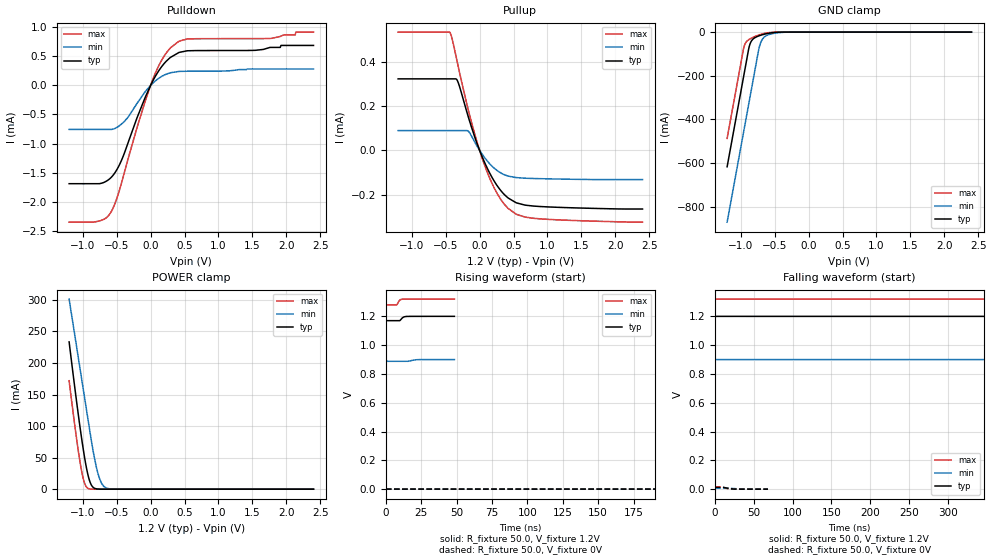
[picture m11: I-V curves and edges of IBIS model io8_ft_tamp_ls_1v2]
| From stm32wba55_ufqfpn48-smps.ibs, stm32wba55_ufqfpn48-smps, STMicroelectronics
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[Model]   io8_ft_tamp_ls_1v2
Model_type I/O
Polarity   Non-Inverting
Enable   Active-Low
| CAP_THRESHOLD on pad IOFT is "UDTCAPC" :
| Rising=30.0% of vddiom   Falling=70.0% of vddiom
| C_comp min and max val. don't necessarily correlate with the min and max pvt
| but are the smallest and greatest pad capacitance found.
| var   typ   min   max
C_comp   4.69416pF  4.27704pF  4.82289pF
|C_comp_pullup   2.95769pF  2.69399pF  2.96399pF
|C_comp_pulldown   1.73647pF  1.58305pF  1.85890pF
Vinl = 450.0mV
Vinh = 660.0mV
Vmeas = 600.0mV   | Reference voltage for timing measurements
Cref  = 50.0pF   | Timing specification test load capacitance value
Rref  = 1.0MOhm   | Timing specification test load resistance value
Vref  = 660.0mV   | Timing specification test load voltage
[Model Spec]
| TIME_THRESHOLD on pin ZIV33SW is "CMOS" :
| Rising=50.0% of VDDV33SW   Falling=50.0% of VDDV33SW
Vinl 436.50000mV 342.50000mV 466.50000mV
Vinh 753.50000mV 549.50000mV 839.50000mV
| variable   typ   min   max
[Temperature Range] 25.0 140.0 -40.0
| variable   typ   min   max
[Voltage Range] 1.2V 900.0mV 1.32V
| variable   typ   min   max
[POWER Clamp Reference] 1.2V 900.0mV 1.32V
| variable   typ   min   max
[GND Clamp Reference] 0V 0V 0V
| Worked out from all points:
|   slope of the pulldown table from 0 to 0.18 V, typ, clamps not added: 517 ohm
|   slope of the pullup table from 0 to 0.18 V, typ, clamps not added: 1.49 kohm
|   GND clamp passes 1 mA (typ) near -0.47 V on its own axis
|   POWER clamp passes 1 mA (typ) near -0.81 V on its own axis
[POWER Clamp]
-1.2V     233.4mA    301.3mA    171.8mA
-1.06V    114.5mA    205.3mA    57.35mA
-1.02V    83.5mA     177.8mA    30.99mA
-980mV    55.21mA    150.4mA    11.87mA
-920mV    21.5mA     109.2mA    1.195mA
-870mV    6.13mA     75.36mA    121.6uA
-820mV    1.189mA    45.7mA     11.82uA
-770mV    199.4uA    22.94mA    1.144uA
-730mV    46.68uA    11.1mA     176.6nA
-680mV    7.557uA    3.666mA    17.16nA
-510mV    15.46nA    46.13uA    134.2pA
2.4V      0A         0A         0A
[GND Clamp]
-1.2V     -616.6mA   -870.4mA   -486.7mA
-960mV    -208.6mA   -462.4mA   -78.75mA
-940mV    -174.6mA   -428.4mA   -56.97mA
-880mV    -73.49mA   -326.4mA   -34.53mA
-850mV    -45.28mA   -275.4mA   -29.09mA
-810mV    -29.66mA   -207.4mA   -23mA
-730mV    -17.09mA   -73.72mA   -13.06mA
-690mV    -13mA      -37.99mA   -9.157mA
-640mV    -8.81mA    -19.57mA   -5.341mA
-520mV    -2.385mA   -6.292mA   -748.7uA
-300mV    -8.501uA   -273.8uA   -150.7nA
2.4V      1.845nA    2.377uA    739.2pA
| variable   typ   min   max
[Pullup Reference] 1.2V 900.0mV 1.32V
| variable   typ   min   max
[Pulldown Reference] 0V 0V 0V
[Pullup]
-1.2V     323uA      89.11uA    534.5uA
-440mV    323uA      89.11uA    534uA
-400mV    323uA      89.11uA    498uA
-340mV    321.5uA    89.11uA    414.8uA
-320mV    310.1uA    89.11uA    386.3uA
-170mV    155.1uA    87.57uA    187.5uA
30mV      -23.17uA   -13.99uA   -28.37uA
220mV     -141.6uA   -81.89uA   -172.9uA
420mV     -215.5uA   -116.5uA   -262.7uA
540mV     -237.3uA   -123.4uA   -289.1uA
790mV     -251.9uA   -127.4uA   -307.1uA
2.4V      -265.4uA   -132.1uA   -324.9uA
[Pulldown]
-1.2V     -1.691mA   -756.9uA   -2.353mA
-760mV    -1.691mA   -756.9uA   -2.334mA
-580mV    -1.582mA   -756.9uA   -2.173mA
-430mV    -1.293mA   -666.3uA   -1.684mA
-200mV    -558.4uA   -310.1uA   -726.5uA
10mV      24.06uA    11.98uA    32.4uA
150mV     302.1uA    144.6uA    405.5uA
290mV     480.2uA    217.1uA    644uA
540mV     595.7uA    243.8uA    798.9uA
1.76V     653.9uA    283.1uA    807.9uA
2.14V     687.4uA    283.1uA    917.2uA
2.4V      687.4uA    283.1uA    917.2uA
[Ramp]
dV/dt_r 7.74127mV/421.4226ns 3.84521mV/812.60829ns 9.4904mV/300.66617ns
dV/dt_f 18.01267mV/399.33434ns 7.33953mV/735.57379ns 24.13809mV/303.15643ns
R_load = 50.0
| Removed startup time: 0s 0s 0s  .
| Removed end time: 48.4ns.
[Rising Waveform]
R_fixture   = 50.0
V_fixture   = 1.2V
V_fixture_min = 900.0mV
V_fixture_max = 1.32V
0s        1.17V      887.8mV    1.28V
7.5ns     1.17V      887.8mV    1.28V
8ns       1.17V      887.8mV    1.284V
9.75ns    1.17V      887.8mV    1.312V
11.7ns    1.19V      887.8mV    1.319V
12.85ns   1.196V     887.8mV    1.32V
15.55ns   1.2V       887.7mV    1.32V
19.9ns    1.2V       896.7mV    1.32V
22.75ns   1.2V       899.2mV    1.32V
48.4ns    1.2V       900mV      1.32V
| Removed startup time: 0s 0s 0s  .
| Removed end time: 4.9984us.
[Falling Waveform]
R_fixture   = 50.0
V_fixture   = 1.2V
V_fixture_min = 900.0mV
V_fixture_max = 1.32V
0s        1.2V       900mV      1.32V
408.1ns   1.2V       900mV      1.319V
510ns     1.199V     900mV      1.313V
581.8ns   1.196V     899.9mV    1.307V
717.6ns   1.189V     899.7mV    1.295V
828.8ns   1.184V     899.1mV    1.288V
1.125us   1.174V     896.1mV    1.281V
1.471us   1.171V     892.3mV    1.28V
2.244us   1.17V      888.4mV    1.28V
4.998us   1.17V      887.8mV    1.28V
| Removed startup time: 0s 0s 0s  .
| Removed end time: 4.9984us.
[Rising Waveform]
R_fixture   = 50.0
V_fixture   = 0V
V_fixture_min = 0V
V_fixture_max = 0V
0s        19.98nV    4.257uV    19.23nV
204ns     -3.458uV   4.106uV    -3.832uV
306.1ns   70.13uV    7.635uV    980.3uV
418ns     1.037mV    20.93uV    4.987mV
614.7ns   5.289mV    126.4uV    11.5mV
797ns     8.764mV    613.8uV    14.35mV
963.6ns   10.79mV    1.443mV    15.33mV
1.306us   12.46mV    3.378mV    15.78mV
2.142us   12.9mV     5.874mV    15.82mV
4.998us   12.9mV     6.413mV    15.82mV
| Removed startup time: 0s 0s 0s  .
| Removed end time: 68.4ns.
[Falling Waveform]
R_fixture   = 50.0
V_fixture   = 0V
V_fixture_min = 0V
V_fixture_max = 0V
0s        12.91mV    6.416mV    15.82mV
8.4ns     12.91mV    6.416mV    15.64mV
11.2ns    12.53mV    6.416mV    11.05mV
15.4ns    7.598mV    6.415mV    4.995mV
18.15ns   4.884mV    6.437mV    2.184mV
20.65ns   2.762mV    5.631mV    858.1uV
24.9ns    752.8uV    3.929mV    202.9uV
31.95ns   109.7uV    1.66mV     55.97uV
37.7ns    45.83uV    586.7uV    16.35uV
68.4ns    286.9nV    16.43uV    734.5nV
